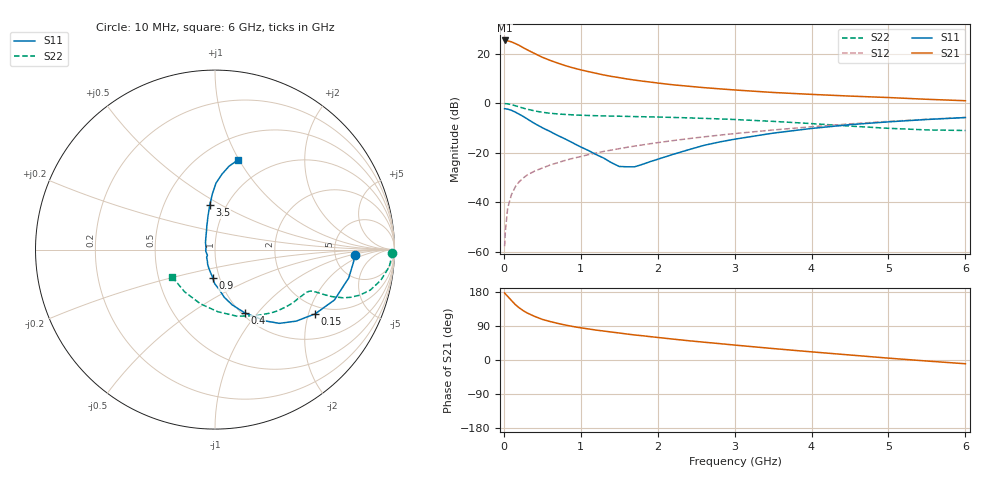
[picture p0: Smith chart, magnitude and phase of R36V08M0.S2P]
! SIEMENS Small Signal Semiconductors
! BFR181
! Si NPN RF Bipolar Junction Transistor in SOT23
! VCE = 6 V  IC = 8 mA
! Common Emitter S-Parameters:  May  1996
# GHz  S  MA  R  50
!  f  S11  S21  S12  S22
! GHz  MAG  ANG  MAG  ANG  MAG  ANG  MAG  ANG
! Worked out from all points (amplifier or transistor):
!   36 points, 10 MHz to 6 GHz, reference 50 ohm
!   highest |S21| = 25.4 dB at 10 MHz (marker M1)
!   |S21| within 3 dB of that: start of sweep to 257.5 MHz
!   unconditionally stable (mu >= 1): 936.7 MHz to 2.793 GHz
!   at 250 MHz: K = 0.53, MSG = 26.4 dB, |S12| = -30.2 dB
!   at 1.4 GHz: K = 1.05, MAG = 13.5 dB, |S12| = -18.9 dB
!   at 6 GHz: K = 0.86, MSG = 3.4 dB, |S12| = -5.7 dB
!   S11 on the Smith chart (normalised r, x): 10 MHz: 7.81, -1.24; 150 MHz: 1.73, -2.21; 400 MHz: 1.03, -0.86; 900 MHz: 0.93, -0.30; 3.5 GHz: 0.84, +0.44; 6 GHz: 0.73, +0.99
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0.01  0.778 -2.3  18.62 176.9  0.0013 89.8  0.9874 -1.0
0.02  0.7757 -4.8  18.36 174.4  0.0026 81.0  0.9847 -2.3
0.05  0.7619 -11.9  18.32 167.9  0.0077 84.5  0.9756 -5.6
0.1  0.7221 -22.9  17.41 156.9  0.0144 80.2  0.9393 -10.5
0.15  0.663 -32.7  16.1 146.0  0.0207 74.3  0.8944 -14.6
0.2  0.6027 -41.4  14.8 137.7  0.026 71.9  0.8449 -17.5
0.25  0.5453 -48.9  13.38 130.5  0.0308 68.8  0.8002 -19.4
0.3  0.4881 -54.6  12.14 124.4  0.0353 68.6  0.7634 -20.6
0.4  0.391 -64.7  10.14 115.1  0.0427 67.1  0.7023 -21.9
0.5  0.3217 -72.8  8.527 107.2  0.0493 67.5  0.6593 -22.4
0.6  0.27 -79.1  7.387 101.6  0.0565 67.4  0.6306 -22.6
0.7  0.2245 -83.9  6.506 96.6  0.0632 67.7  0.6104 -22.8
0.9  0.1577 -94.4  5.201 88.3  0.0775 67.9  0.5845 -23.3
1.1  0.1113 -107.6  4.367 82.0  0.0919 68.2  0.5676 -24.5
1.3  0.078 -122.8  3.737 76.4  0.1068 68.0  0.5569 -25.9
1.6  0.0522 -170.1  3.105 68.5  0.129 67.2  0.5445 -28.8
2.2  0.0931 122.4  2.366 55.1  0.1766 64.3  0.5186 -36.1
2.8  0.1651 104.7  1.964 43.3  0.227 60.1  0.4849 -45.1
3.5  0.2498 96.7  1.657 30.2  0.2893 54.2  0.4319 -58.8
4.5  0.3709 89.1  1.4 13.2  0.3844 43.6  0.3465 -87.4
5.5  0.4716 80.4  1.206 -2.7  0.4763 31.1  0.29 -125.8
6  0.5159 75.6  1.128 -9.9  0.5186 24.2  0.2826 -147.5
